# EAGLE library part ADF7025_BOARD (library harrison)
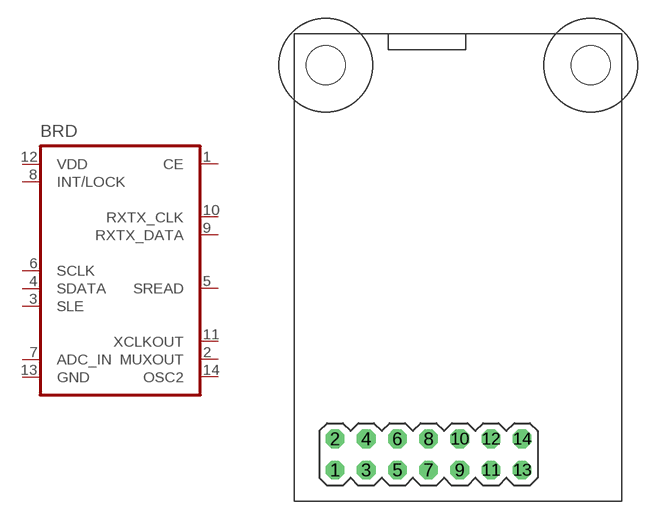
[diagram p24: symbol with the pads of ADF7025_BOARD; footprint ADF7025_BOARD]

Designator prefix BRD

## ADF7025_BOARD  [ADF7025_BOARD]
1  CE  in
2  MUXOUT  out
3  SLE  in
4  SDATA  in
5  SREAD  out
6  SCLK  in
7  ADC_IN  in
8  INT/LOCK
9  RXTX_DATA  out
10  RXTX_CLK  out
11  XCLKOUT  out
12  VDD  pwr
13  GND  pwr
14  OSC2  out

## Footprint ADF7025_BOARD (pad centres in mm)
drill 1.016 octagon: 1 3.302,2.54; 2 3.302,5.08; 3 5.842,2.54; 4 5.842,5.08; 5 8.382,2.54; 6 8.382,5.08; 7 10.922,2.54; 8 10.922,5.08; 9 13.462,2.54; 10 13.462,5.08; 11 16.002,2.54; 12 16.002,5.08; 13 18.542,2.54; 14 18.542,5.08
hole 3.2 at 2.54,35.56
hole 3.2 at 24.13,35.56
